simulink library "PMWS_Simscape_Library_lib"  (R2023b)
settings: Solver=VariableStepAuto  StartTime=0.0  StopTime=10.0  RelTol=1e-3
undefined symbols (not defined in the file or in its folder): A, Battery, Brake, compiletime, DifferentialGear, Engine, gcbh, GearBox, Input_angle, kg, lambda_method_tire, m, Motor, N, Ohm, plane_source, PlanetaryGear, PMWS_Simscape_Library, rad, rpm, s, simscape, Steering, TorqueConverter, V, Vehicle, Vehicle_3DoF

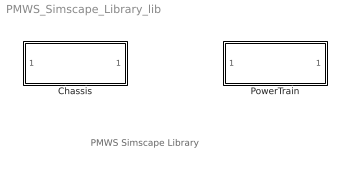
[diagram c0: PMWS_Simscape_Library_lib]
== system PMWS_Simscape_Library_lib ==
  note: PMWS Simscape Library
  Chassis : Subsystem  Tag=simscape_sublibrary
  PowerTrain : Subsystem  Tag=simscape_sublibrary

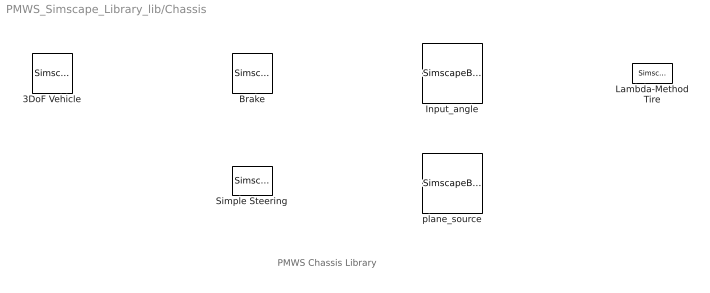
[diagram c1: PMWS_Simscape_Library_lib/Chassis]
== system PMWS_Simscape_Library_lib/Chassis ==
  note: PMWS Chassis Library
  3DoF Vehicle : SimscapeBlock  DialogController=NetworkEngine.DynNeDlgSource  LoadFcn=simscape.compiler.sli.internal.callback('LoadFcn',gcbh);  SourceFile=PMWS_Simscape_Library.Chassis.Vehicle_3DoF  mask(3DoF Vehicle){ComponentPath=PMWS_Simscape_Library.Chassis.Vehicle_3DoF, ComponentVariants=["PMWS_Simscape_Library.Chassis.Vehicle_3DoF"], ComponentVariantNames=["Vehicle_3DoF"], ClassName=Vehicle_3DoF, SchemaVersion=1, m=1500, m_unit=kg, m_conf=compiletime, g=9.81, g_unit=m/s^2, g_conf=compiletime, I=2e3, I_unit=kg*m^2, I_conf=compiletime, lf=1.8, lf_unit=m, lf_conf=compiletime, lr=2.4, lr_unit=m, lr_conf=compiletime, wrl=1, wrl_unit=m, wrl_conf=compiletime, Af=3, Af_unit=m^2, Af_conf=compiletime, Cd=0.4, Cd_unit=1, Cd_conf=compiletime, rho=1.2, rho_unit=kg/m^3, rho_conf=compiletime, D_1=0.01, D_1_unit=kg/s, D_1_conf=compiletime, D_2=0.01, D_2_unit=kg/s, D_2_conf=compiletime, D_3=0.01, D_3_unit=N*m*s, D_3_conf=compiletime, Fx1_specify=off, Fx1_priority=None, Fx1=0.0, Fx1_unit=N, Fx1_nominal_specify=off, Fx1_nominal_unit=N, Fx1_nominal_value=1, Fx2_specify=off, Fx2_priority=None, Fx2=0.0, Fx2_unit=N, Fx2_nominal_specify=off, Fx2_nominal_unit=N, Fx2_nominal_value=1, Fx3_specify=off, Fx3_priority=None, Fx3=0.0, Fx3_unit=N, Fx3_nominal_specify=off, Fx3_nominal_unit=N, Fx3_nominal_value=1, Fx4_specify=off, Fx4_priority=None, Fx4=0.0, Fx4_unit=N, Fx4_nominal_specify=off, Fx4_nominal_unit=N, Fx4_nominal_value=1, Fy1_specify=off, Fy1_priority=None, Fy1=0.0, Fy1_unit=N, Fy1_nominal_specify=off, Fy1_nominal_unit=N, Fy1_nominal_value=1, Fy2_specify=off, Fy2_priority=None, Fy2=0.0, Fy2_unit=N, Fy2_nominal_specify=off, Fy2_nominal_unit=N, Fy2_nominal_value=1, Fy3_specify=off, Fy3_priority=None, Fy3=0.0, Fy3_unit=N, Fy3_nominal_specify=off, Fy3_nominal_unit=N, Fy3_nominal_value=1, Fy4_specify=off, Fy4_priority=None, Fy4=0.0, Fy4_unit=N, Fy4_nominal_specify=off, Fy4_nominal_unit=N, Fy4_nominal_value=1, Mz_specify=off, Mz_priority=None, Mz=0.0, Mz_unit=N*m, Mz_nominal_specify=off, Mz_nominal_unit=N*m, Mz_nominal_value=1, Omega_specify=off, Omega_priority=None, Omega=0.0, Omega_unit=rad/s, Omega_nominal_specify=off, Omega_nominal_unit=rad/s, Omega_nominal_value=1, Px1_specify=off, Px1_priority=None, Px1=1.0, Px1_unit=m, Px1_nominal_specify=off, Px1_nominal_unit=m, Px1_nominal_value=1, Px2_specify=off, Px2_priority=None, Px2=1.0, Px2_unit=m, Px2_nominal_specify=off, Px2_nominal_unit=m, Px2_nominal_value=1, Px3_specify=off, Px3_priority=None, Px3=1.0, Px3_unit=m, Px3_nominal_specify=off, Px3_nominal_unit=m, Px3_nominal_value=1, Px4_specify=off, Px4_priority=None, Px4=1.0, Px4_unit=m, Px4_nominal_specify=off, Px4_nominal_unit=m, Px4_nominal_value=1, Py1_specify=off, Py1_priority=None, Py1=1.0, Py1_unit=m, Py1_nominal_specify=off, Py1_nominal_unit=m, Py1_nominal_value=1, Py2_specify=off, Py2_priority=None, Py2=1.0, Py2_unit=m, Py2_nominal_specify=off, Py2_nominal_unit=m, Py2_nominal_value=1, Py3_specify=off, Py3_priority=None, Py3=1.0, Py3_unit=m, Py3_nominal_specify=off, Py3_nominal_unit=m, Py3_nominal_value=1, Py4_specify=off, Py4_priority=None, Py4=1.0, Py4_unit=m, Py4_nominal_specify=off, Py4_nominal_unit=m, Py4_nominal_value=1, OP1_specify=off, OP1_priority=None, OP1=1.0, OP1_unit=m, OP1_nominal_specify=off, OP1_nominal_unit=m, OP1_nominal_value=1, OP2_specify=off, OP2_priority=None, OP2=1.0, OP2_unit=m, OP2_nominal_specify=off, OP2_nominal_unit=m, OP2_nominal_value=1, OP3_specify=off, OP3_priority=None, OP3=1.0, OP3_unit=m, OP3_nominal_specify=off, OP3_nominal_unit=m, OP3_nominal_value=1, OP4_specify=off, OP4_priority=None, OP4=1.0, OP4_unit=m, OP4_nominal_specify=off, OP4_nominal_unit=m, OP4_nominal_value=1, phi1_specify=off, phi1_priority=None, phi1=0.0, phi1_unit=rad, phi1_nominal_specify=off, phi1_nominal_unit=rad, phi1_nominal_value=1, phi2_specify=off, phi2_priority=None, phi2=0.0, phi2_unit=rad, phi2_nominal_specify=off, phi2_nominal_unit=rad, phi2_nominal_value=1, phi3_specify=off, phi3_priority=None, phi3=0.0, phi3_unit=rad, phi3_nominal_specify=off, phi3_nominal_unit=rad, phi3_nominal_value=1, phi4_specify=off, phi4_priority=None, phi4=0.0, phi4_unit=rad, phi4_nominal_specify=off, phi4_nominal_unit=rad, phi4_nominal_value=1, vx_wcs_specify=off, vx_wcs_priority=None, vx_wcs=0.0, vx_wcs_unit=m/s, vx_wcs_nominal_specify=off, vx_wcs_nominal_unit=m/s, vx_wcs_nominal_value=1, vy_wcs_specify=off, vy_wcs_priority=None, vy_wcs=0.0, vy_wcs_unit=m/s, vy_wcs_nominal_specify=off, vy_wcs_nominal_unit=m/s, vy_wcs_nominal_value=1, yaw_specify=off, yaw_priority=None, yaw=0.0, yaw_unit=rad, yaw_nominal_specify=off, yaw_nominal_unit=rad, yaw_nominal_value=1}
      mask prompts: m "Mass"; I "Inertia"; lf "From G to Front"; lr "From G to Rear"; wrl "From G to Right/Left"; Af "Frontal area"; Cd "Drag coefficient"; rho "Atmospheric air density"; Fx1_specify "Fx1"; Fx1_priority "Fx1"; Fx1_nominal_specify "Fx1"; Fx2_specify "Fx2"; Fx2_priority "Fx2"; Fx2_nominal_specify "Fx2"; Fx3_specify "Fx3"; Fx3_priority "Fx3"; Fx3_nominal_specify "Fx3"; Fx4_specify "Fx4"; Fx4_priority "Fx4"; Fx4_nominal_specify "Fx4"; Fy1_specify "Fy1"; Fy1_priority "Fy1"; Fy1_nominal_specify "Fy1"; Fy2_specify "Fy2"; Fy2_priority "Fy2"; Fy2_nominal_specify "Fy2"; Fy3_specify "Fy3"; Fy3_priority "Fy3"; Fy3_nominal_specify "Fy3"; Fy4_specify "Fy4"; Fy4_priority "Fy4"; Fy4_nominal_specify "Fy4"; Mz_specify "Mz"; Mz_priority "Mz"; Mz_nominal_specify "Mz"; Omega_specify "Omega"; Omega_priority "Omega"; Omega_nominal_specify "Omega"; Px1_specify "Px1"; Px1_priority "Px1"; Px1_nominal_specify "Px1"; Px2_specify "Px2"; Px2_priority "Px2"; Px2_nominal_specify "Px2"; Px3_specify "Px3"; Px3_priority "Px3"; Px3_nominal_specify "Px3"; Px4_specify "Px4"; Px4_priority "Px4"; Px4_nominal_specify "Px4"; Py1_specify "Py1"; Py1_priority "Py1"; Py1_nominal_specify "Py1"; Py2_specify "Py2"; Py2_priority "Py2"; Py2_nominal_specify "Py2"; Py3_specify "Py3"; Py3_priority "Py3"; Py3_nominal_specify "Py3"; Py4_specify "Py4"; Py4_priority "Py4"; Py4_nominal_specify "Py4"; OP1_specify "OP1"; OP1_priority "OP1"; OP1_nominal_specify "OP1"; OP2_specify "OP2"; OP2_priority "OP2"; OP2_nominal_specify "OP2"; OP3_specify "OP3"; OP3_priority "OP3"; OP3_nominal_specify "OP3"; OP4_specify "OP4"; OP4_priority "OP4"; OP4_nominal_specify "OP4"; phi1_specify "phi1"; phi1_priority "phi1"; phi1_nominal_specify "phi1"; phi2_specify "phi2"; phi2_priority "phi2"; phi2_nominal_specify "phi2"; phi3_specify "phi3"; phi3_priority "phi3"; phi3_nominal_specify "phi3"; phi4_specify "phi4"; phi4_priority "phi4"; phi4_nominal_specify "phi4"; vx_wcs_specify "vx_wcs"; vx_wcs_priority "vx_wcs"; vx_wcs_nominal_specify "vx_wcs"; vy_wcs_specify "vy_wcs"; vy_wcs_priority "vy_wcs"; vy_wcs_nominal_specify "vy_wcs"; yaw_specify "yaw"; yaw_priority "yaw"; yaw_nominal_specify "yaw"
      mask help: Ver. 1.0 Jun/22, 2017 JMAAB Plant Modeling Workshop
      mask init:
      | simscape.compiler.sli.internal.preinitmask(gcb);
  Brake : SimscapeBlock  DialogController=NetworkEngine.DynNeDlgSource  LoadFcn=simscape.compiler.sli.internal.callback('LoadFcn',gcbh);  SourceFile=PMWS_Simscape_Library.Chassis.Brake  mask(Brake){ComponentPath=PMWS_Simscape_Library.Chassis.Brake, ComponentVariants=["PMWS_Simscape_Library.Chassis.Brake"], ComponentVariantNames=["Brake"], ClassName=Brake, SchemaVersion=1, w_thr=3.0, w_thr_unit=rad/s, w_thr_conf=compiletime, Brake_force_thr=0.1, Brake_force_thr_unit=N, Brake_force_thr_conf=compiletime, T_L=1.0, T_L_unit=s, T_L_conf=compiletime, uk=1.0, uk_unit=1, uk_conf=compiletime, Er=1.0, Er_unit=m, Er_conf=compiletime, w_T_specify=off, w_T_priority=None, w_T=0, w_T_unit=rad/s, w_T_nominal_specify=off, w_T_nominal_unit=rad/s, w_T_nominal_value=1, t_F_specify=off, t_F_priority=None, t_F=0, t_F_unit=N*m, t_F_nominal_specify=off, t_F_nominal_unit=N*m, t_F_nominal_value=1, t_T_specify=off, t_T_priority=None, t_T=0, t_T_unit=N*m, t_T_nominal_specify=off, t_T_nominal_unit=N*m, t_T_nominal_value=1, state_specify=off, state_priority=None, state=0, state_unit=1, state_nominal_specify=off, state_nominal_unit=1, state_nominal_value=1}
      mask prompts: uk "Kinetic friction coefficient"; Er "Effective radius"; w_T_specify "w_T"; w_T_priority "w_T"; w_T_nominal_specify "w_T"; t_F_specify "t_F"; t_F_priority "t_F"; t_F_nominal_specify "t_F"; t_T_specify "t_T"; t_T_priority "t_T"; t_T_nominal_specify "t_T"; state_specify "state"; state_priority "state"; state_nominal_specify "state"
      mask help: Ver. 1.0 Jun/22, 2017 JMAAB Plant Modeling Workshop
      mask init:
      | simscape.compiler.sli.internal.preinitmask(gcb);
  Input_angle : SimscapeBlock  DialogController=NetworkEngine.DynNeDlgSource  LoadFcn=simscape.compiler.sli.internal.callback('LoadFcn',gcbh);  SourceFile=PMWS_Simscape_Library.Chassis.Input_angle  mask(Input_angle){ComponentPath=PMWS_Simscape_Library.Chassis.Input_angle, ComponentVariants=["PMWS_Simscape_Library.Chassis.Input_angle"], ComponentVariantNames=["Input_angle"], ClassName=Input_angle, SchemaVersion=1, delta=0, delta_unit=rad, delta_conf=compiletime, Mz_specify=off, Mz_priority=None, Mz=0.0, Mz_unit=N*m, Mz_nominal_specify=off, Mz_nominal_unit=N*m, Mz_nominal_value=1}
      mask prompts: Mz_specify "Mz"; Mz_priority "Mz"; Mz_nominal_specify "Mz"
      mask help: Ver. 1.0 Jun/22, 2017 JMAAB Plant Modeling Workshop
      mask init:
      | simscape.compiler.sli.internal.preinitmask(gcb);
  Lambda-Method Tire : SimscapeBlock  DialogController=NetworkEngine.DynNeDlgSource  LoadFcn=simscape.compiler.sli.internal.callback('LoadFcn',gcbh);  SourceFile=PMWS_Simscape_Library.Chassis.lambda_method_tire  mask(Lambda-Method Tire){ComponentPath=PMWS_Simscape_Library.Chassis.lambda_method_tire, ComponentVariants=["PMWS_Simscape_Library.Chassis.lambda_method_tire"], ComponentVariantNames=["lambda_method_tire"], ClassName=lambda_method_tire, SchemaVersion=1, c_1=1.0, c_1_unit=1, c_1_conf=compiletime, c_2=30.0, c_2_unit=1, c_2_conf=compiletime, c_3=2.0, c_3_unit=1, c_3_conf=compiletime, I=1, I_unit=kg*m^2, I_conf=compiletime, R=0.3, R_unit=m, R_conf=compiletime, epsiv=1e-6, epsiv_unit=1, epsiv_conf=compiletime, eps_lambda=0.000001, eps_lambda_unit=1, eps_lambda_conf=compiletime, V_X_specify=off, V_X_priority=None, V_X=0.0, V_X_unit=m/s, V_X_nominal_specify=off, V_X_nominal_unit=m/s, V_X_nominal_value=1, V_Y_specify=off, V_Y_priority=None, V_Y=0.0, V_Y_unit=m/s, V_Y_nominal_specify=off, V_Y_nominal_unit=m/s, V_Y_nominal_value=1, V_specify=off, V_priority=None, V=0.0, V_unit=m/s, V_nominal_specify=off, V_nominal_unit=m/s, V_nominal_value=1, V_omega_specify=off, V_omega_priority=None, V_omega=0.0, V_omega_unit=m/s, V_omega_nominal_specify=off, V_omega_nominal_unit=m/s, V_omega_nominal_value=1, maxV_specify=off, maxV_priority=None, maxV=0.001, maxV_unit=m/s, maxV_nominal_specify=off, maxV_nominal_unit=m/s, maxV_nominal_value=1, delta_specify=off, delta_priority=None, delta=0, delta_unit=rad, delta_nominal_specify=off, delta_nominal_unit=rad, delta_nominal_value=1, lambda_specify=off, lambda_priority=None, lambda=0.0, lambda_unit=1, lambda_nominal_specify=off, lambda_nominal_unit=1, lambda_nominal_value=1, lambda_x_specify=off, lambda_x_priority=None, lambda_x=0.0, lambda_x_unit=1, lambda_x_nominal_specify=off, lambda_x_nominal_unit=1, lambda_x_nominal_value=1, abs_lambda_x_specify=off, abs_lambda_x_priority=None, abs_lambda_x=0.0, abs_lambda_x_unit=1, abs_lambda_x_nominal_specify=off, abs_lambda_x_nominal_unit=1, abs_lambda_x_nominal_value=1, lambda_y_specify=off, lambda_y_priority=None, lambda_y=0.0, lambda_y_unit=1, lambda_y_nominal_specify=off, lambda_y_nominal_unit=1, lambda_y_nominal_value=1, abs_lambda_y_specify=off, abs_lambda_y_priority=None, abs_lambda_y=0.0, abs_lambda_y_unit=1, abs_lambda_y_nominal_specify=off, abs_lambda_y_nominal_unit=1, abs_lambda_y_nominal_value=1, lambda_angle_specify=off, lambda_angle_priority=None, lambda_angle=0.0, lambda_angle_unit=rad, lambda_angle_nominal_specify=off, lambda_angle_nominal_unit=rad, lambda_angle_nominal_value=1, mu_specify=off, mu_priority=None, mu=0.0, mu_unit=1, mu_nominal_specify=off, mu_nominal_unit=1, mu_nominal_value=1, mu_x_specify=off, mu_x_priority=None, mu_x=0.0, mu_x_unit=1, mu_x_nominal_specify=off, mu_x_nominal_unit=1, mu_x_nominal_value=1, mu_y_specify=off, mu_y_priority=None, mu_y=0.0, mu_y_unit=1, mu_y_nominal_specify=off, mu_y_nominal_unit=1, mu_y_nominal_value=1, f_x_specify=off, f_x_priority=None, f_x=0.0, f_x_unit=N, f_x_nominal_specify=off, f_x_nominal_unit=N, f_x_nominal_value=1, f_y_specify=off, f_y_priority=None, f_y=0.0, f_y_unit=N, f_y_nominal_specify=off, f_y_nominal_unit=N, f_y_nominal_value=1, Fx_specify=off, Fx_priority=None, Fx=0.0, Fx_unit=N, Fx_nominal_specify=off, Fx_nominal_unit=N, Fx_nominal_value=1, Fy_specify=off, Fy_priority=None, Fy=0.0, Fy_unit=N, Fy_nominal_specify=off, Fy_nominal_unit=N, Fy_nominal_value=1, Mz_specify=off, Mz_priority=None, Mz=0.0, Mz_unit=N*m, Mz_nominal_specify=off, Mz_nominal_unit=N*m, Mz_nominal_value=1, Tin_specify=off, Tin_priority=None, Tin=0.0, Tin_unit=N*m, Tin_nominal_specify=off, Tin_nominal_unit=N*m, Tin_nominal_value=1}
      mask prompts: I "Inertia"; R "Radius"; V_X_specify "V_X"; V_X_priority "V_X"; V_X_nominal_specify "V_X"; V_Y_specify "V_Y"; V_Y_priority "V_Y"; V_Y_nominal_specify "V_Y"; V_specify "V"; V_priority "V"; V_nominal_specify "V"; V_omega_specify "V_omega"; V_omega_priority "V_omega"; V_omega_nominal_specify "V_omega"; maxV_specify "maxV"; maxV_priority "maxV"; maxV_nominal_specify "maxV"; delta_specify "delta"; delta_priority "delta"; delta_nominal_specify "delta"; lambda_specify "lambda"; lambda_priority "lambda"; lambda_nominal_specify "lambda"; lambda_x_specify "lambda_x"; lambda_x_priority "lambda_x"; lambda_x_nominal_specify "lambda_x"; abs_lambda_x_specify "abs_lambda_x"; abs_lambda_x_priority "abs_lambda_x"; abs_lambda_x_nominal_specify "abs_lambda_x"; lambda_y_specify "lambda_y"; lambda_y_priority "lambda_y"; lambda_y_nominal_specify "lambda_y"; abs_lambda_y_specify "abs_lambda_y"; abs_lambda_y_priority "abs_lambda_y"; abs_lambda_y_nominal_specify "abs_lambda_y"; lambda_angle_specify "lambda_angle"; lambda_angle_priority "lambda_angle"; lambda_angle_nominal_specify "lambda_angle"; mu_specify "mu"; mu_priority "mu"; mu_nominal_specify "mu"; mu_x_specify "mu_x"; mu_x_priority "mu_x"; mu_x_nominal_specify "mu_x"; mu_y_specify "mu_y"; mu_y_priority "mu_y"; mu_y_nominal_specify "mu_y"; f_x_specify "f_x"; f_x_priority "f_x"; f_x_nominal_specify "f_x"; f_y_specify "f_y"; f_y_priority "f_y"; f_y_nominal_specify "f_y"; Fx_specify "Fx"; Fx_priority "Fx"; Fx_nominal_specify "Fx"; Fy_specify "Fy"; Fy_priority "Fy"; Fy_nominal_specify "Fy"; Mz_specify "Mz"; Mz_priority "Mz"; Mz_nominal_specify "Mz"; Tin_specify "Tin"; Tin_priority "Tin"; Tin_nominal_specify "Tin"
      mask help: Ver. 1.0 Jun/22, 2017 JMAAB Plant Modeling Workshop
      mask init:
      | simscape.compiler.sli.internal.preinitmask(gcb);
  Simple Steering : SimscapeBlock  DialogController=NetworkEngine.DynNeDlgSource  LoadFcn=simscape.compiler.sli.internal.callback('LoadFcn',gcbh);  SourceFile=PMWS_Simscape_Library.Chassis.Steering  mask(Simple Steering){ComponentPath=PMWS_Simscape_Library.Chassis.Steering, ComponentVariants=["PMWS_Simscape_Library.Chassis.Steering"], ComponentVariantNames=["Steering"], ClassName=Steering, SchemaVersion=1, ratio=1 / 16, ratio_unit=1, ratio_conf=compiletime, Mz_L_specify=off, Mz_L_priority=None, Mz_L=0.0, Mz_L_unit=N*m, Mz_L_nominal_specify=off, Mz_L_nominal_unit=N*m, Mz_L_nominal_value=1, Mz_R_specify=off, Mz_R_priority=None, Mz_R=0.0, Mz_R_unit=N*m, Mz_R_nominal_specify=off, Mz_R_nominal_unit=N*m, Mz_R_nominal_value=1}
      mask prompts: ratio "Gear ratio"; Mz_L_specify "Mz_L"; Mz_L_priority "Mz_L"; Mz_L_nominal_specify "Mz_L"; Mz_R_specify "Mz_R"; Mz_R_priority "Mz_R"; Mz_R_nominal_specify "Mz_R"
      mask help: Ver. 1.0 Jun/22, 2017 JMAAB Plant Modeling Workshop
      mask init:
      | simscape.compiler.sli.internal.preinitmask(gcb);
  plane_source : SimscapeBlock  DialogController=NetworkEngine.DynNeDlgSource  LoadFcn=simscape.compiler.sli.internal.callback('LoadFcn',gcbh);  SourceFile=PMWS_Simscape_Library.Chassis.plane_source  mask(plane_source){ComponentPath=PMWS_Simscape_Library.Chassis.plane_source, ComponentVariants=["PMWS_Simscape_Library.Chassis.plane_source"], ComponentVariantNames=["plane_source"], ClassName=plane_source, SchemaVersion=1, Fx_specify=off, Fx_priority=None, Fx=0.0, Fx_unit=N, Fx_nominal_specify=off, Fx_nominal_unit=N, Fx_nominal_value=1, Fy_specify=off, Fy_priority=None, Fy=0.0, Fy_unit=N, Fy_nominal_specify=off, Fy_nominal_unit=N, Fy_nominal_value=1}
      mask prompts: Fx_specify "Fx"; Fx_priority "Fx"; Fx_nominal_specify "Fx"; Fy_specify "Fy"; Fy_priority "Fy"; Fy_nominal_specify "Fy"
      mask help: Ver. 1.0 Jun/22, 2017 JMAAB Plant Modeling Workshop
      mask init:
      | simscape.compiler.sli.internal.preinitmask(gcb);

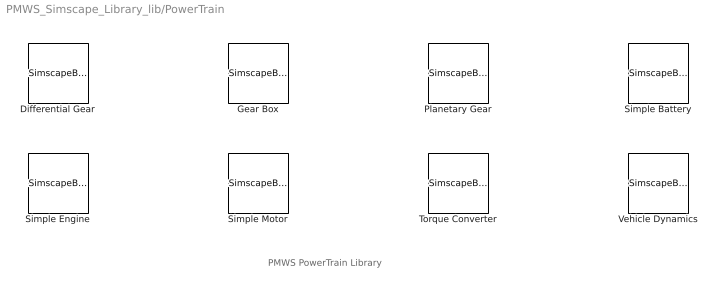
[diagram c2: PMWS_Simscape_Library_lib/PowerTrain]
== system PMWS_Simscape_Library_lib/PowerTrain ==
  note: PMWS PowerTrain Library
  Differential Gear : SimscapeBlock  DialogController=NetworkEngine.DynNeDlgSource  LoadFcn=simscape.compiler.sli.internal.callback('LoadFcn',gcbh);  SourceFile=PMWS_Simscape_Library.PowerTrain.DifferentialGear  mask(Differential Gear){ComponentPath=PMWS_Simscape_Library.PowerTrain.DifferentialGear, ComponentVariants=["PMWS_Simscape_Library.PowerTrain.DifferentialGear"], ComponentVariantNames=["DifferentialGear"], ClassName=DifferentialGear, SchemaVersion=1, Eta=0.9, Eta_unit=1, Eta_conf=compiletime, Rin=1.33, Rin_unit=1, Rin_conf=compiletime, Rps=1, Rps_unit=1, Rps_conf=compiletime, Ip=0.01, Ip_unit=kg*m^2, Ip_conf=compiletime, t_in_specify=off, t_in_priority=None, t_in=0, t_in_unit=N*m, t_in_nominal_specify=off, t_in_nominal_unit=N*m, t_in_nominal_value=1, t_out1_specify=off, t_out1_priority=None, t_out1=0, t_out1_unit=N*m, t_out1_nominal_specify=off, t_out1_nominal_unit=N*m, t_out1_nominal_value=1, t_out2_specify=off, t_out2_priority=None, t_out2=0, t_out2_unit=N*m, t_out2_nominal_specify=off, t_out2_nominal_unit=N*m, t_out2_nominal_value=1, w_in_specify=off, w_in_priority=None, w_in=0, w_in_unit=rad/s, w_in_nominal_specify=off, w_in_nominal_unit=rad/s, w_in_nominal_value=1, w_s1_specify=off, w_s1_priority=None, w_s1=0, w_s1_unit=rad/s, w_s1_nominal_specify=off, w_s1_nominal_unit=rad/s, w_s1_nominal_value=1, w_s2_specify=off, w_s2_priority=None, w_s2=0, w_s2_unit=rad/s, w_s2_nominal_specify=off, w_s2_nominal_unit=rad/s, w_s2_nominal_value=1, w_p_specify=off, w_p_priority=None, w_p=0, w_p_unit=rad/s, w_p_nominal_specify=off, w_p_nominal_unit=rad/s, w_p_nominal_value=1}
      mask prompts: Eta "Eta : Differential Gear Efficiency"; Rin "Rin : Ring(Follower) Gear to Input(base) Gear teeth ratio (NF/NB)"; Rps "Rps : Pion(Planet) Gear to Side(sun) Gear teeth ratio (NP/NS)"; Ip "Ip : Pinionn Gear Inertia"; t_in_specify "t_in"; t_in_priority "t_in"; t_in_nominal_specify "t_in"; t_out1_specify "t_out1"; t_out1_priority "t_out1"; t_out1_nominal_specify "t_out1"; t_out2_specify "t_out2"; t_out2_priority "t_out2"; t_out2_nominal_specify "t_out2"; w_in_specify "w_in"; w_in_priority "w_in"; w_in_nominal_specify "w_in"; w_s1_specify "w_s1"; w_s1_priority "w_s1"; w_s1_nominal_specify "w_s1"; w_s2_specify "w_s2"; w_s2_priority "w_s2"; w_s2_nominal_specify "w_s2"; w_p_specify "w_p"; w_p_priority "w_p"; w_p_nominal_specify "w_p"
      mask help: Ver. 1.0 Jun/22, 2017 JMAAB Plant Modeling Workshop
      mask init:
      | simscape.compiler.sli.internal.preinitmask(gcb);
  Gear Box : SimscapeBlock  DialogController=NetworkEngine.DynNeDlgSource  LoadFcn=simscape.compiler.sli.internal.callback('LoadFcn',gcbh);  SourceFile=PMWS_Simscape_Library.PowerTrain.GearBox  mask(Gear Box){ComponentPath=PMWS_Simscape_Library.PowerTrain.GearBox, ComponentVariants=["PMWS_Simscape_Library.PowerTrain.GearBox"], ComponentVariantNames=["GearBox"], ClassName=GearBox, SchemaVersion=1, kp=1 / 3e+5, kp_unit=N*m/rad, kp_conf=compiletime, kv=1 / 0.05, kv_unit=N*m*s/rad, kv_conf=compiletime, T_in_specify=off, T_in_priority=None, T_in=0, T_in_unit=N*m, T_in_nominal_specify=off, T_in_nominal_unit=N*m, T_in_nominal_value=1, T_out_specify=off, T_out_priority=None, T_out=0, T_out_unit=N*m, T_out_nominal_specify=off, T_out_nominal_unit=N*m, T_out_nominal_value=1, W_in_specify=off, W_in_priority=None, W_in=0, W_in_unit=rad/s, W_in_nominal_specify=off, W_in_nominal_unit=rad/s, W_in_nominal_value=1, W_out_specify=off, W_out_priority=None, W_out=0, W_out_unit=rad/s, W_out_nominal_specify=off, W_out_nominal_unit=rad/s, W_out_nominal_value=1, ph_specify=off, ph_priority=None, ph=0, ph_unit=rad, ph_nominal_specify=off, ph_nominal_unit=rad, ph_nominal_value=1, dph_specify=off, dph_priority=None, dph=0, dph_unit=rad/s, dph_nominal_specify=off, dph_nominal_unit=rad/s, dph_nominal_value=1}
      mask prompts: kp "Base/input angular compliance (kp)"; kv "Base/input angular compliance damping (kv)"; T_in_specify "T_in"; T_in_priority "T_in"; T_in_nominal_specify "T_in"; T_out_specify "T_out"; T_out_priority "T_out"; T_out_nominal_specify "T_out"; W_in_specify "W_in"; W_in_priority "W_in"; W_in_nominal_specify "W_in"; W_out_specify "W_out"; W_out_priority "W_out"; W_out_nominal_specify "W_out"; ph_specify "ph"; ph_priority "ph"; ph_nominal_specify "ph"; dph_specify "dph"; dph_priority "dph"; dph_nominal_specify "dph"
      mask help: Ver. 1.0 Jun/22, 2017 JMAAB Plant Modeling Workshop
      mask init:
      | simscape.compiler.sli.internal.preinitmask(gcb);
  Planetary Gear : SimscapeBlock  DialogController=NetworkEngine.DynNeDlgSource  LoadFcn=simscape.compiler.sli.internal.callback('LoadFcn',gcbh);  SourceFile=PMWS_Simscape_Library.PowerTrain.PlanetaryGear  mask(Planetary Gear){ComponentPath=PMWS_Simscape_Library.PowerTrain.PlanetaryGear, ComponentVariants=["PMWS_Simscape_Library.PowerTrain.PlanetaryGear"], ComponentVariantNames=["PlanetaryGear"], ClassName=PlanetaryGear, SchemaVersion=1, Zs=1, Zs_unit=1, Zs_conf=compiletime, Zr=1, Zr_unit=1, Zr_conf=compiletime, tc_specify=off, tc_priority=None, tc=0, tc_unit=N*m, tc_nominal_specify=off, tc_nominal_unit=N*m, tc_nominal_value=1, tr_specify=off, tr_priority=None, tr=0, tr_unit=N*m, tr_nominal_specify=off, tr_nominal_unit=N*m, tr_nominal_value=1, ts_specify=off, ts_priority=None, ts=0, ts_unit=N*m, ts_nominal_specify=off, ts_nominal_unit=N*m, ts_nominal_value=1, wc_specify=off, wc_priority=None, wc=0, wc_unit=rad/s, wc_nominal_specify=off, wc_nominal_unit=rad/s, wc_nominal_value=1, wr_specify=off, wr_priority=None, wr=0, wr_unit=rad/s, wr_nominal_specify=off, wr_nominal_unit=rad/s, wr_nominal_value=1, ws_specify=off, ws_priority=None, ws=0, ws_unit=rad/s, ws_nominal_specify=off, ws_nominal_unit=rad/s, ws_nominal_value=1, gr_specify=off, gr_priority=None, gr=1, gr_unit=1, gr_nominal_specify=off, gr_nominal_unit=1, gr_nominal_value=1}
      mask prompts: Zs "Sun gear Teeth Number"; Zr "Ring gear Teeth Number"; tc_specify "tc"; tc_priority "tc"; tc_nominal_specify "tc"; tr_specify "tr"; tr_priority "tr"; tr_nominal_specify "tr"; ts_specify "ts"; ts_priority "ts"; ts_nominal_specify "ts"; wc_specify "wc"; wc_priority "wc"; wc_nominal_specify "wc"; wr_specify "wr"; wr_priority "wr"; wr_nominal_specify "wr"; ws_specify "ws"; ws_priority "ws"; ws_nominal_specify "ws"; gr_specify "gr"; gr_priority "gr"; gr_nominal_specify "gr"
      mask help: Ver. 1.0 Jun/22, 2017 JMAAB Plant Modeling Workshop
      mask init:
      | simscape.compiler.sli.internal.preinitmask(gcb);
  Simple Battery : SimscapeBlock  DialogController=NetworkEngine.DynNeDlgSource  LoadFcn=simscape.compiler.sli.internal.callback('LoadFcn',gcbh);  SourceFile=PMWS_Simscape_Library.PowerTrain.Battery  mask(Simple Battery){ComponentPath=PMWS_Simscape_Library.PowerTrain.Battery, ComponentVariants=["PMWS_Simscape_Library.PowerTrain.Battery"], ComponentVariantNames=["Battery"], ClassName=Battery, SchemaVersion=1, SOC_init=60, SOC_init_unit=1, SOC_init_conf=compiletime, Qmax=7 * 3600, Qmax_unit=A*s, Qmax_conf=compiletime, R=0.1, R_unit=Ohm, R_conf=compiletime, Ib_specify=off, Ib_priority=None, Ib=0, Ib_unit=A, Ib_nominal_specify=off, Ib_nominal_unit=A, Ib_nominal_value=1, Vb_specify=off, Vb_priority=None, Vb=0, Vb_unit=V, Vb_nominal_specify=off, Vb_nominal_unit=V, Vb_nominal_value=1, Q_internal_specify=off, Q_internal_priority=None, Q_internal=0, Q_internal_unit=A*s, Q_internal_nominal_specify=off, Q_internal_nominal_unit=A*s, Q_internal_nominal_value=1, Q_current_specify=off, Q_current_priority=None, Q_current=0, Q_current_unit=A*s, Q_current_nominal_specify=off, Q_current_nominal_unit=A*s, Q_current_nominal_value=1}
      mask prompts: SOC_init "Initial SOC [%]"; Qmax "Max Capacity"; R "Internal Resisitance"; Ib_specify "Ib"; Ib_priority "Ib"; Ib_nominal_specify "Ib"; Vb_specify "Vb"; Vb_priority "Vb"; Vb_nominal_specify "Vb"; Q_internal_specify "Q_internal"; Q_internal_priority "Q_internal"; Q_internal_nominal_specify "Q_internal"; Q_current_specify "Q_current"; Q_current_priority "Q_current"; Q_current_nominal_specify "Q_current"
      mask help: Ver. 1.0 Jun/22, 2017 JMAAB Plant Modeling Workshop
      mask init:
      | simscape.compiler.sli.internal.preinitmask(gcb);
  Simple Engine : SimscapeBlock  DialogController=NetworkEngine.DynNeDlgSource  LoadFcn=simscape.compiler.sli.internal.callback('LoadFcn',gcbh);  SourceFile=PMWS_Simscape_Library.PowerTrain.Engine  mask(Simple Engine){ComponentPath=PMWS_Simscape_Library.PowerTrain.Engine, ComponentVariants=["PMWS_Simscape_Library.PowerTrain.Engine"], ComponentVariantNames=["Engine"], ClassName=Engine, SchemaVersion=1, Rev=[0, 500, 1000, 2000, 3000, 4000], Rev_unit=rpm, Rev_conf=compiletime, Torque=[200, 400, 400, 400, 400, 400], Torque_unit=N*m, Torque_conf=compiletime, interp_method=1, interp_method_unit=1, interp_method_conf=compiletime, extrap_method=2, extrap_method_unit=1, extrap_method_conf=compiletime, Te_specify=off, Te_priority=None, Te=0, Te_unit=N*m, Te_nominal_specify=off, Te_nominal_unit=N*m, Te_nominal_value=1, W_specify=off, W_priority=None, W=0, W_unit=rad/s, W_nominal_specify=off, W_nominal_unit=rad/s, W_nominal_value=1}
      mask prompts: Rev "Vector of engine speed"; Torque "Vector of max engine torque"; interp_method "Interpolation method"; extrap_method "Extrapolation method"; Te_specify "Te"; Te_priority "Te"; Te_nominal_specify "Te"; W_specify "W"; W_priority "W"; W_nominal_specify "W"
      mask help: Ver. 1.0 Jun/22, 2017 JMAAB Plant Modeling Workshop
      mask init:
      | simscape.compiler.sli.internal.preinitmask(gcb);
  Simple Motor : SimscapeBlock  DialogController=NetworkEngine.DynNeDlgSource  LoadFcn=simscape.compiler.sli.internal.callback('LoadFcn',gcbh);  SourceFile=PMWS_Simscape_Library.PowerTrain.Motor  mask(Simple Motor){ComponentPath=PMWS_Simscape_Library.PowerTrain.Motor, ComponentVariants=["PMWS_Simscape_Library.PowerTrain.Motor"], ComponentVariantNames=["Motor"], ClassName=Motor, SchemaVersion=1, Efficiency=0.9, Efficiency_unit=1, Efficiency_conf=compiletime, I_max=300, I_max_unit=A, I_max_conf=compiletime, I_specify=off, I_priority=None, I=0, I_unit=A, I_nominal_specify=off, I_nominal_unit=A, I_nominal_value=1, I_temp_specify=off, I_temp_priority=None, I_temp=0, I_temp_unit=A, I_temp_nominal_specify=off, I_temp_nominal_unit=A, I_temp_nominal_value=1, V_specify=off, V_priority=None, V=0, V_unit=V, V_nominal_specify=off, V_nominal_unit=V, V_nominal_value=1, T_specify=off, T_priority=None, T=0, T_unit=N*m, T_nominal_specify=off, T_nominal_unit=N*m, T_nominal_value=1, W_specify=off, W_priority=None, W=0, W_unit=rad/s, W_nominal_specify=off, W_nominal_unit=rad/s, W_nominal_value=1}
      mask prompts: Efficiency "Motor efficiency"; I_max "Max motor current"; I_specify "I"; I_priority "I"; I_nominal_specify "I"; I_temp_specify "I_temp"; I_temp_priority "I_temp"; I_temp_nominal_specify "I_temp"; V_specify "V"; V_priority "V"; V_nominal_specify "V"; T_specify "T"; T_priority "T"; T_nominal_specify "T"; W_specify "W"; W_priority "W"; W_nominal_specify "W"
      mask help: Ver. 1.0 Jun/22, 2017 JMAAB Plant Modeling Workshop
      mask init:
      | simscape.compiler.sli.internal.preinitmask(gcb);
  Torque Converter : SimscapeBlock  DialogController=NetworkEngine.DynNeDlgSource  LoadFcn=simscape.compiler.sli.internal.callback('LoadFcn',gcbh);  SourceFile=PMWS_Simscape_Library.PowerTrain.TorqueConverter  mask(Torque Converter){ComponentPath=PMWS_Simscape_Library.PowerTrain.TorqueConverter, ComponentVariants=["PMWS_Simscape_Library.PowerTrain.TorqueConverter"], ComponentVariantNames=["TorqueConverter"], ClassName=TorqueConverter, SchemaVersion=1, SpeedRatio_th=0.97, SpeedRatio_th_unit=1, SpeedRatio_th_conf=compiletime, K_th=50.00, K_th_unit=rad/(N^(1/2)*m^(1/2)*s), K_th_conf=compiletime, W_th=0.1 * (2 * pi) / 60, W_th_unit=rad/s, W_th_conf=compiletime, T_impeller_specify=off, T_impeller_priority=None, T_impeller=0, T_impeller_unit=N*m, T_impeller_nominal_specify=off, T_impeller_nominal_unit=N*m, T_impeller_nominal_value=1, T_turbine_specify=off, T_turbine_priority=None, T_turbine=0, T_turbine_unit=N*m, T_turbine_nominal_specify=off, T_turbine_nominal_unit=N*m, T_turbine_nominal_value=1, W_impeller_specify=off, W_impeller_priority=None, W_impeller=0, W_impeller_unit=rad/s, W_impeller_nominal_specify=off, W_impeller_nominal_unit=rad/s, W_impeller_nominal_value=1, W_turbine_specify=off, W_turbine_priority=None, W_turbine=0, W_turbine_unit=rad/s, W_turbine_nominal_specify=off, W_turbine_nominal_unit=rad/s, W_turbine_nominal_value=1}
      mask prompts: SpeedRatio_th "Threshold (Speed Ratio)"; K_th "Threshold (Capacitify Factor)"; W_th "Threshold (Angular Speed)"; T_impeller_specify "T_impeller"; T_impeller_priority "T_impeller"; T_impeller_nominal_specify "T_impeller"; T_turbine_specify "T_turbine"; T_turbine_priority "T_turbine"; T_turbine_nominal_specify "T_turbine"; W_impeller_specify "W_impeller"; W_impeller_priority "W_impeller"; W_impeller_nominal_specify "W_impeller"; W_turbine_specify "W_turbine"; W_turbine_priority "W_turbine"; W_turbine_nominal_specify "W_turbine"
      mask help: Ver. 1.0 Jun/22, 2017 JMAAB Plant Modeling Workshop
      mask init:
      | simscape.compiler.sli.internal.preinitmask(gcb);
  Vehicle Dynamics : SimscapeBlock  DialogController=NetworkEngine.DynNeDlgSource  LoadFcn=simscape.compiler.sli.internal.callback('LoadFcn',gcbh);  SourceFile=PMWS_Simscape_Library.PowerTrain.Vehicle  mask(Vehicle Dynamics){ComponentPath=PMWS_Simscape_Library.PowerTrain.Vehicle, ComponentVariants=["PMWS_Simscape_Library.PowerTrain.Vehicle"], ComponentVariantNames=["Vehicle"], ClassName=Vehicle, SchemaVersion=1, m=1200.00, m_unit=kg, m_conf=compiletime, nt=2.00, nt_unit=1, nt_conf=compiletime, a=1.40, a_unit=m, a_conf=compiletime, b=1.60, b_unit=m, b_conf=compiletime, h=0.50, h_unit=m, h_conf=compiletime, Af=3.00, Af_unit=m^2, Af_conf=compiletime, Cd=0.40, Cd_unit=1, Cd_conf=compiletime, v0=0.00, v0_unit=m/s, v0_conf=compiletime, rho=1.20, rho_unit=kg/m^3, rho_conf=compiletime, g=9.81, g_unit=m/s^2, g_conf=compiletime, Fxt_specify=off, Fxt_priority=None, Fxt=0, Fxt_unit=N, Fxt_nominal_specify=off, Fxt_nominal_unit=N, Fxt_nominal_value=1, Vx_specify=off, Vx_priority=None, Vx=0, Vx_unit=m/s, Vx_nominal_specify=off, Vx_nominal_unit=m/s, Vx_nominal_value=1, Fd_specify=off, Fd_priority=None, Fd=0, Fd_unit=N, Fd_nominal_specify=off, Fd_nominal_unit=N, Fd_nominal_value=1, Fa_specify=off, Fa_priority=None, Fa=0, Fa_unit=N, Fa_nominal_specify=off, Fa_nominal_unit=N, Fa_nominal_value=1, Fzf_specify=off, Fzf_priority=None, Fzf=0, Fzf_unit=N, Fzf_nominal_specify=off, Fzf_nominal_unit=N, Fzf_nominal_value=1, Fzr_specify=off, Fzr_priority=None, Fzr=0, Fzr_unit=N, Fzr_nominal_specify=off, Fzr_nominal_unit=N, Fzr_nominal_value=1}
      mask prompts: m "Vehicle mass"; nt "Number of wheels on each axle"; a "Distance of front axle, respectively, from the normal projection point of vehicle CG onto the common axle plane"; b "Distance of rear axle, respectively, from the normal projection point of vehicle CG onto the common axle plane"; h "CG height above ground"; Af "Effective frontal vehicle cross-sectional area"; Cd "Aerodynamic drag coefficient"; v0 "Initial velocity"; rho "Mass density of air"; g "Gravitational acceleration"; Fxt_specify "Fxt"; Fxt_priority "Fxt"; Fxt_nominal_specify "Fxt"; Vx_specify "Vx"; Vx_priority "Vx"; Vx_nominal_specify "Vx"; Fd_specify "Fd"; Fd_priority "Fd"; Fd_nominal_specify "Fd"; Fa_specify "Fa"; Fa_priority "Fa"; Fa_nominal_specify "Fa"; Fzf_specify "Fzf"; Fzf_priority "Fzf"; Fzf_nominal_specify "Fzf"; Fzr_specify "Fzr"; Fzr_priority "Fzr"; Fzr_nominal_specify "Fzr"
      mask help: Ver. 1.0 Jun/22, 2017 JMAAB Plant Modeling Workshop
      mask init:
      | simscape.compiler.sli.internal.preinitmask(gcb);
